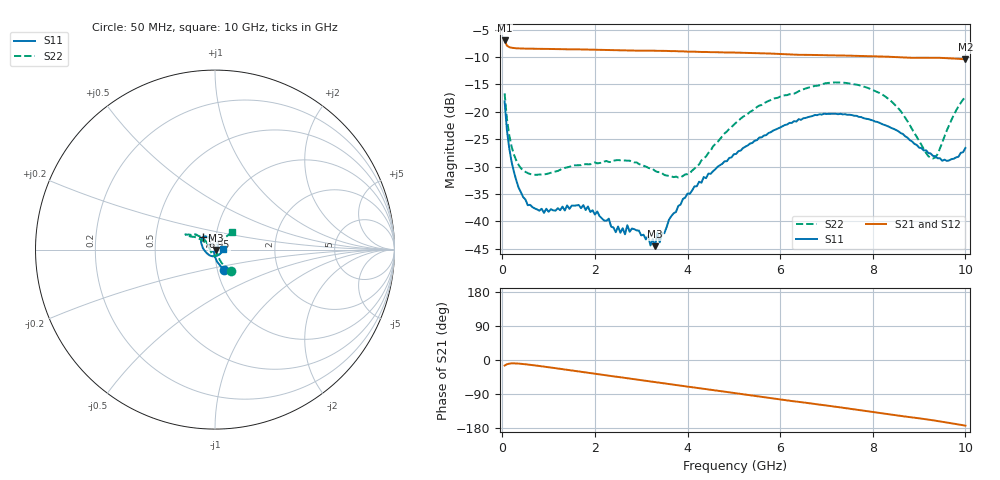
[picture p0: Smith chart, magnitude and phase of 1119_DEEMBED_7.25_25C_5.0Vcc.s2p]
!Hittite Microwave Corp.
!Digital Attenuator/PhaseShifter Rev 1.4.0
!Filename: C:\DATA\DATA\1119_DEEMBED_7.25_25C_5.0Vcc.s2p
!VNA ID: Agilent Technologies,N5224A,MY51441122,A.10.45.03
!Device type:
!2 Port Calibration.
!Temp(C): 25
!Lot Number:
!Serial Number:
!Operator:
!Misc:
!Attenuator:  7.250
# GHZ S DB R 50.0
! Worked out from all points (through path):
!   200 points, 50 MHz to 10 GHz, reference 50 ohm
!   highest |S21| = -6.98 dB at 50 MHz (marker M1); lowest = -10.4 dB at 10 GHz (marker M2)
!   group delay of S21, straight-line fit = 46.6 ps
!   lowest |S11| = -44.5 dB at 3.3 GHz (marker M3), VSWR 1.01, Z = 50.5 - j0.277 ohm
!   |S11| at or under -10 dB: start of sweep to end of sweep
!   |S22| runs from -32.0 to -14.6 dB; largest |S21 - S12| = 0.0013
!   S11 on the Smith chart (normalised r, x): 50 MHz: 1.07, -0.25; 6.95 GHz: 0.87, +0.12; 10 GHz: 1.10, +0.00
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0.05  -18.11 -67.0  -6.98 -14.7  -6.98 -14.7  -16.64 -53.5
0.15  -26.64 -87.2  -8.20 -9.5  -8.20 -9.5  -24.27 -65.3
0.25  -30.92 -95.3  -8.37 -8.8  -8.38 -8.8  -27.81 -64.3
0.55  -37.07 -112.8  -8.48 -11.9  -8.47 -11.9  -31.21 -59.6
0.9  -38.48 -122.9  -8.52 -17.4  -8.52 -17.4  -31.43 -62.7
1.75  -37.05 -123.9  -8.62 -31.8  -8.62 -31.8  -29.60 -78.9
2.3  -39.53 -114.9  -8.72 -41.3  -8.72 -41.4  -29.18 -93.3
2.45  -42.00 -101.8  -8.77 -43.9  -8.78 -44.0  -28.88 -97.3
2.65  -42.38 -88.8  -8.82 -47.2  -8.82 -47.3  -28.91 -104.0
2.7  -40.73 -79.4  -8.82 -48.0  -8.82 -48.1  -28.94 -104.8
3.3  -44.55 -27.6  -8.87 -58.1  -8.87 -58.2  -30.81 -129.0
3.35  -42.09 -14.8  -8.87 -59.0  -8.88 -59.0  -31.00 -130.5
3.4  -43.85 -14.7  -8.87 -59.8  -8.88 -59.9  -31.04 -133.0
3.6  -39.70 14.0  -8.92 -63.5  -8.93 -63.5  -31.73 -142.7
4.05  -34.98 33.9  -9.01 -71.0  -9.02 -71.1  -31.20 179.6
5.05  -27.70 80.5  -9.20 -87.8  -9.21 -87.8  -21.98 136.4
6.7  -20.78 128.2  -9.63 -115.2  -9.64 -115.3  -15.39 150.2
6.95  -20.35 132.8  -9.68 -119.2  -9.69 -119.2  -14.86 152.3
8.35  -22.74 166.1  -9.96 -143.2  -9.96 -143.2  -17.73 147.7
9.3  -28.05 -113.3  -10.13 -159.1  -10.15 -159.2  -28.54 107.1
9.65  -28.88 -55.0  -10.23 -166.0  -10.24 -166.0  -22.41 52.7
10  -26.62 1.6  -10.43 -173.2  -10.44 -173.1  -17.28 46.0
